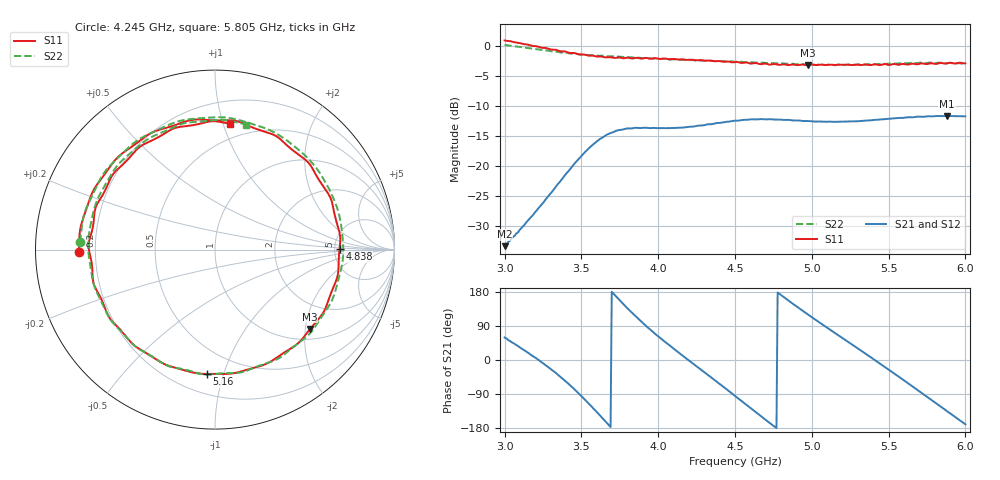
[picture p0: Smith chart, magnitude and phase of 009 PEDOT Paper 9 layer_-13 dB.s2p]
!  04/11/2025  20:01:51
! Ref Plane: 0.000 mm
# MHZ S MA R  50
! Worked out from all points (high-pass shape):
!   401 points, 3 GHz to 6 GHz, reference 50 ohm
!   highest |S21| = -11.67 dB at 5.88 GHz (marker M1); lowest = -33.3 dB at 3 GHz (marker M2)
!   |S21| within 3 dB of the highest: 3.675 GHz to end of sweep
!   lowest |S11| = -3.2 dB at 4.973 GHz (marker M3), VSWR 5.45, Z = 62.7 - j106 ohm
!   |S11| at or under -10 dB: nowhere
!   |S22| runs from -3.2 to 0.2 dB; largest |S21 - S12| = 0.0069
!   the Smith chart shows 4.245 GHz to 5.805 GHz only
!   S11 on the Smith chart (normalised r, x): 4.245 GHz: 0.14, -0.01; 4.838 GHz: 5.53, +0.10; 5.16 GHz: 0.33, -0.88; 5.805 GHz: 0.38, +1.06
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3000  1.107 -115.0  0.02153 59.3  0.02168 60.8  1.018 -119.1
3142.5  1.027 -149.0  0.03414 21.9  0.03406 23.2  0.96 -152.5
3270  0.9579 177.7  0.05335 -14.3  0.05324 -12.8  0.916 173.6
3390  0.8981 140.4  0.08292 -53.3  0.08323 -52.6  0.8785 135.4
3502.5  0.8478 98.5  0.1223 -96.2  0.1224 -95.5  0.846 92.8
3637.5  0.8105 41.4  0.1726 -153.8  0.1735 -153.0  0.8268 35.3
3735  0.798 -2.2  0.1979 163.6  0.1981 164.8  0.8121 -7.2
3870  0.7923 -56.9  0.2073 108.7  0.2087 109.9  0.7963 -61.5
4005  0.7775 -104.5  0.2064 61.0  0.206 62.0  0.7765 -108.4
4245  0.7579 -179.1  0.2145 -15.2  0.2152 -13.7  0.7531 176.7
4500  0.7326 103.0  0.2381 -94.9  0.2394 -93.9  0.7363 95.4
4687.5  0.7099 44.9  0.2447 -154.2  0.2446 -153.3  0.7218 33.8
4837.5  0.6939 0.4  0.242 160.0  0.2414 161.1  0.7076 -13.8
4972.5  0.6898 -39.9  0.2366 120.7  0.2362 121.8  0.6978 -54.4
5002.5  0.6975 -48.6  0.2349 112.5  0.2344 113.4  0.6997 -62.4
5160  0.6942 -93.7  0.233 68.6  0.2329 69.5  0.6913 -106.8
5347.5  0.7001 -146.6  0.2384 17.3  0.2385 18.1  0.6972 -156.6
5505  0.6921 169.0  0.2471 -26.6  0.2481 -25.3  0.711 160.4
5655  0.7098 126.1  0.2541 -69.6  0.2548 -68.2  0.7195 118.6
5805  0.7061 83.0  0.2599 -113.1  0.2613 -111.7  0.7185 75.9
5880  0.7125 61.1  0.2609 -135.0  0.2621 -133.8  0.7191 54.2
6000  0.7137 28.1  0.2589 -169.7  0.2596 -168.7  0.706 19.9
